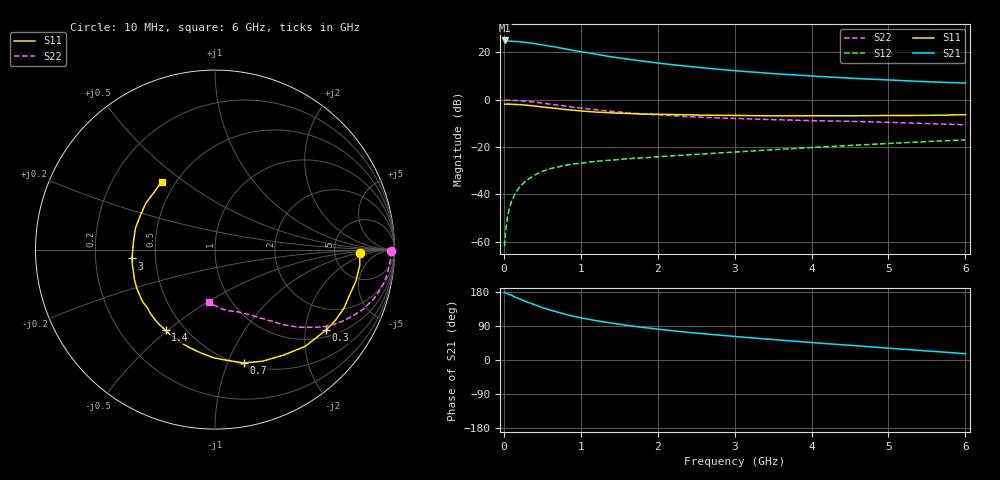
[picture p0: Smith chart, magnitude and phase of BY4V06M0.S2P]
! SIEMENS Small Signal Semiconductors
! BFY420
! Si NPN RF SIEGET Grounded Emitter Transistor in MICRO-X
! VCE = 4 V  IC = 6 mA
! Common Emitter S-Parameters:  October  1996
# GHz  S  MA  R  50
!  f  S11  S21  S12  S22
! GHz  MAG  ANG  MAG  ANG  MAG  ANG  MAG  ANG
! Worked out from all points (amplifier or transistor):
!   36 points, 10 MHz to 6 GHz, reference 50 ohm
!   highest |S21| = 25.1 dB at 10 MHz (marker M1)
!   |S21| within 3 dB of that: start of sweep to 705.6 MHz
!   unconditionally stable (mu >= 1): 2.984 GHz to end of sweep
!   at 250 MHz: K = 0.18, MSG = 29.9 dB, |S12| = -35.3 dB
!   at 1.4 GHz: K = 0.59, MSG = 21.9 dB, |S12| = -25.6 dB
!   at 6 GHz: K = 1.12, MAG = 9.9 dB, |S12| = -17.0 dB
!   S11 on the Smith chart (normalised r, x): 10 MHz: 9.20, -1.03; 300 MHz: 1.20, -2.59; 700 MHz: 0.52, -1.15; 1.4 GHz: 0.40, -0.49; 3 GHz: 0.37, -0.05; 6 GHz: 0.42, +0.41
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0.01  0.8061 -1.4  17.94 179.4  0.0008 45.5  0.9817 -0.5
0.02  0.8062 -2.5  17.76 177.3  0.0015 51.2  0.9765 -1.1
0.05  0.8117 -6.0  17.4 174.5  0.0037 71.6  0.9805 -2.9
0.1  0.8047 -12.6  17.31 170.9  0.0071 75.8  0.9732 -5.9
0.15  0.7918 -18.4  17.02 165.5  0.0105 75.4  0.9664 -8.8
0.2  0.7894 -24.2  16.89 162.0  0.014 74.0  0.9578 -11.5
0.3  0.7641 -35.9  16.17 153.2  0.02 70.0  0.928 -17.0
0.4  0.7371 -47.0  15.42 146.0  0.0256 65.8  0.8909 -21.8
0.5  0.7009 -57.0  14.45 138.1  0.0304 61.1  0.8492 -26.0
0.7  0.6517 -75.6  12.75 126.2  0.0377 55.1  0.7714 -33.1
0.9  0.6017 -91.1  11.08 115.6  0.0438 50.4  0.6986 -38.3
1.1  0.5632 -105.1  9.808 107.6  0.048 47.4  0.6394 -42.6
1.2  0.5491 -111.1  9.186 103.8  0.0497 46.5  0.6133 -44.3
1.4  0.5265 -121.5  8.075 97.4  0.0527 44.5  0.5712 -47.3
1.6  0.5131 -131.1  7.252 91.4  0.0564 43.1  0.5323 -49.9
1.8  0.4966 -139.7  6.574 86.2  0.0588 42.8  0.503 -52.1
2.2  0.4864 -153.3  5.482 77.1  0.0652 41.2  0.4598 -56.3
3  0.4652 -173.9  4.12 62.1  0.0783 40.6  0.4029 -63.4
3.5  0.4564 174.9  3.569 53.9  0.0877 39.1  0.3795 -67.6
4.5  0.4575 155.3  2.857 38.7  0.1078 35.6  0.35 -77.0
5.5  0.4664 136.4  2.403 24.0  0.1305 29.9  0.3131 -89.5
6  0.4814 128.2  2.251 16.7  0.1419 26.5  0.2952 -97.0
